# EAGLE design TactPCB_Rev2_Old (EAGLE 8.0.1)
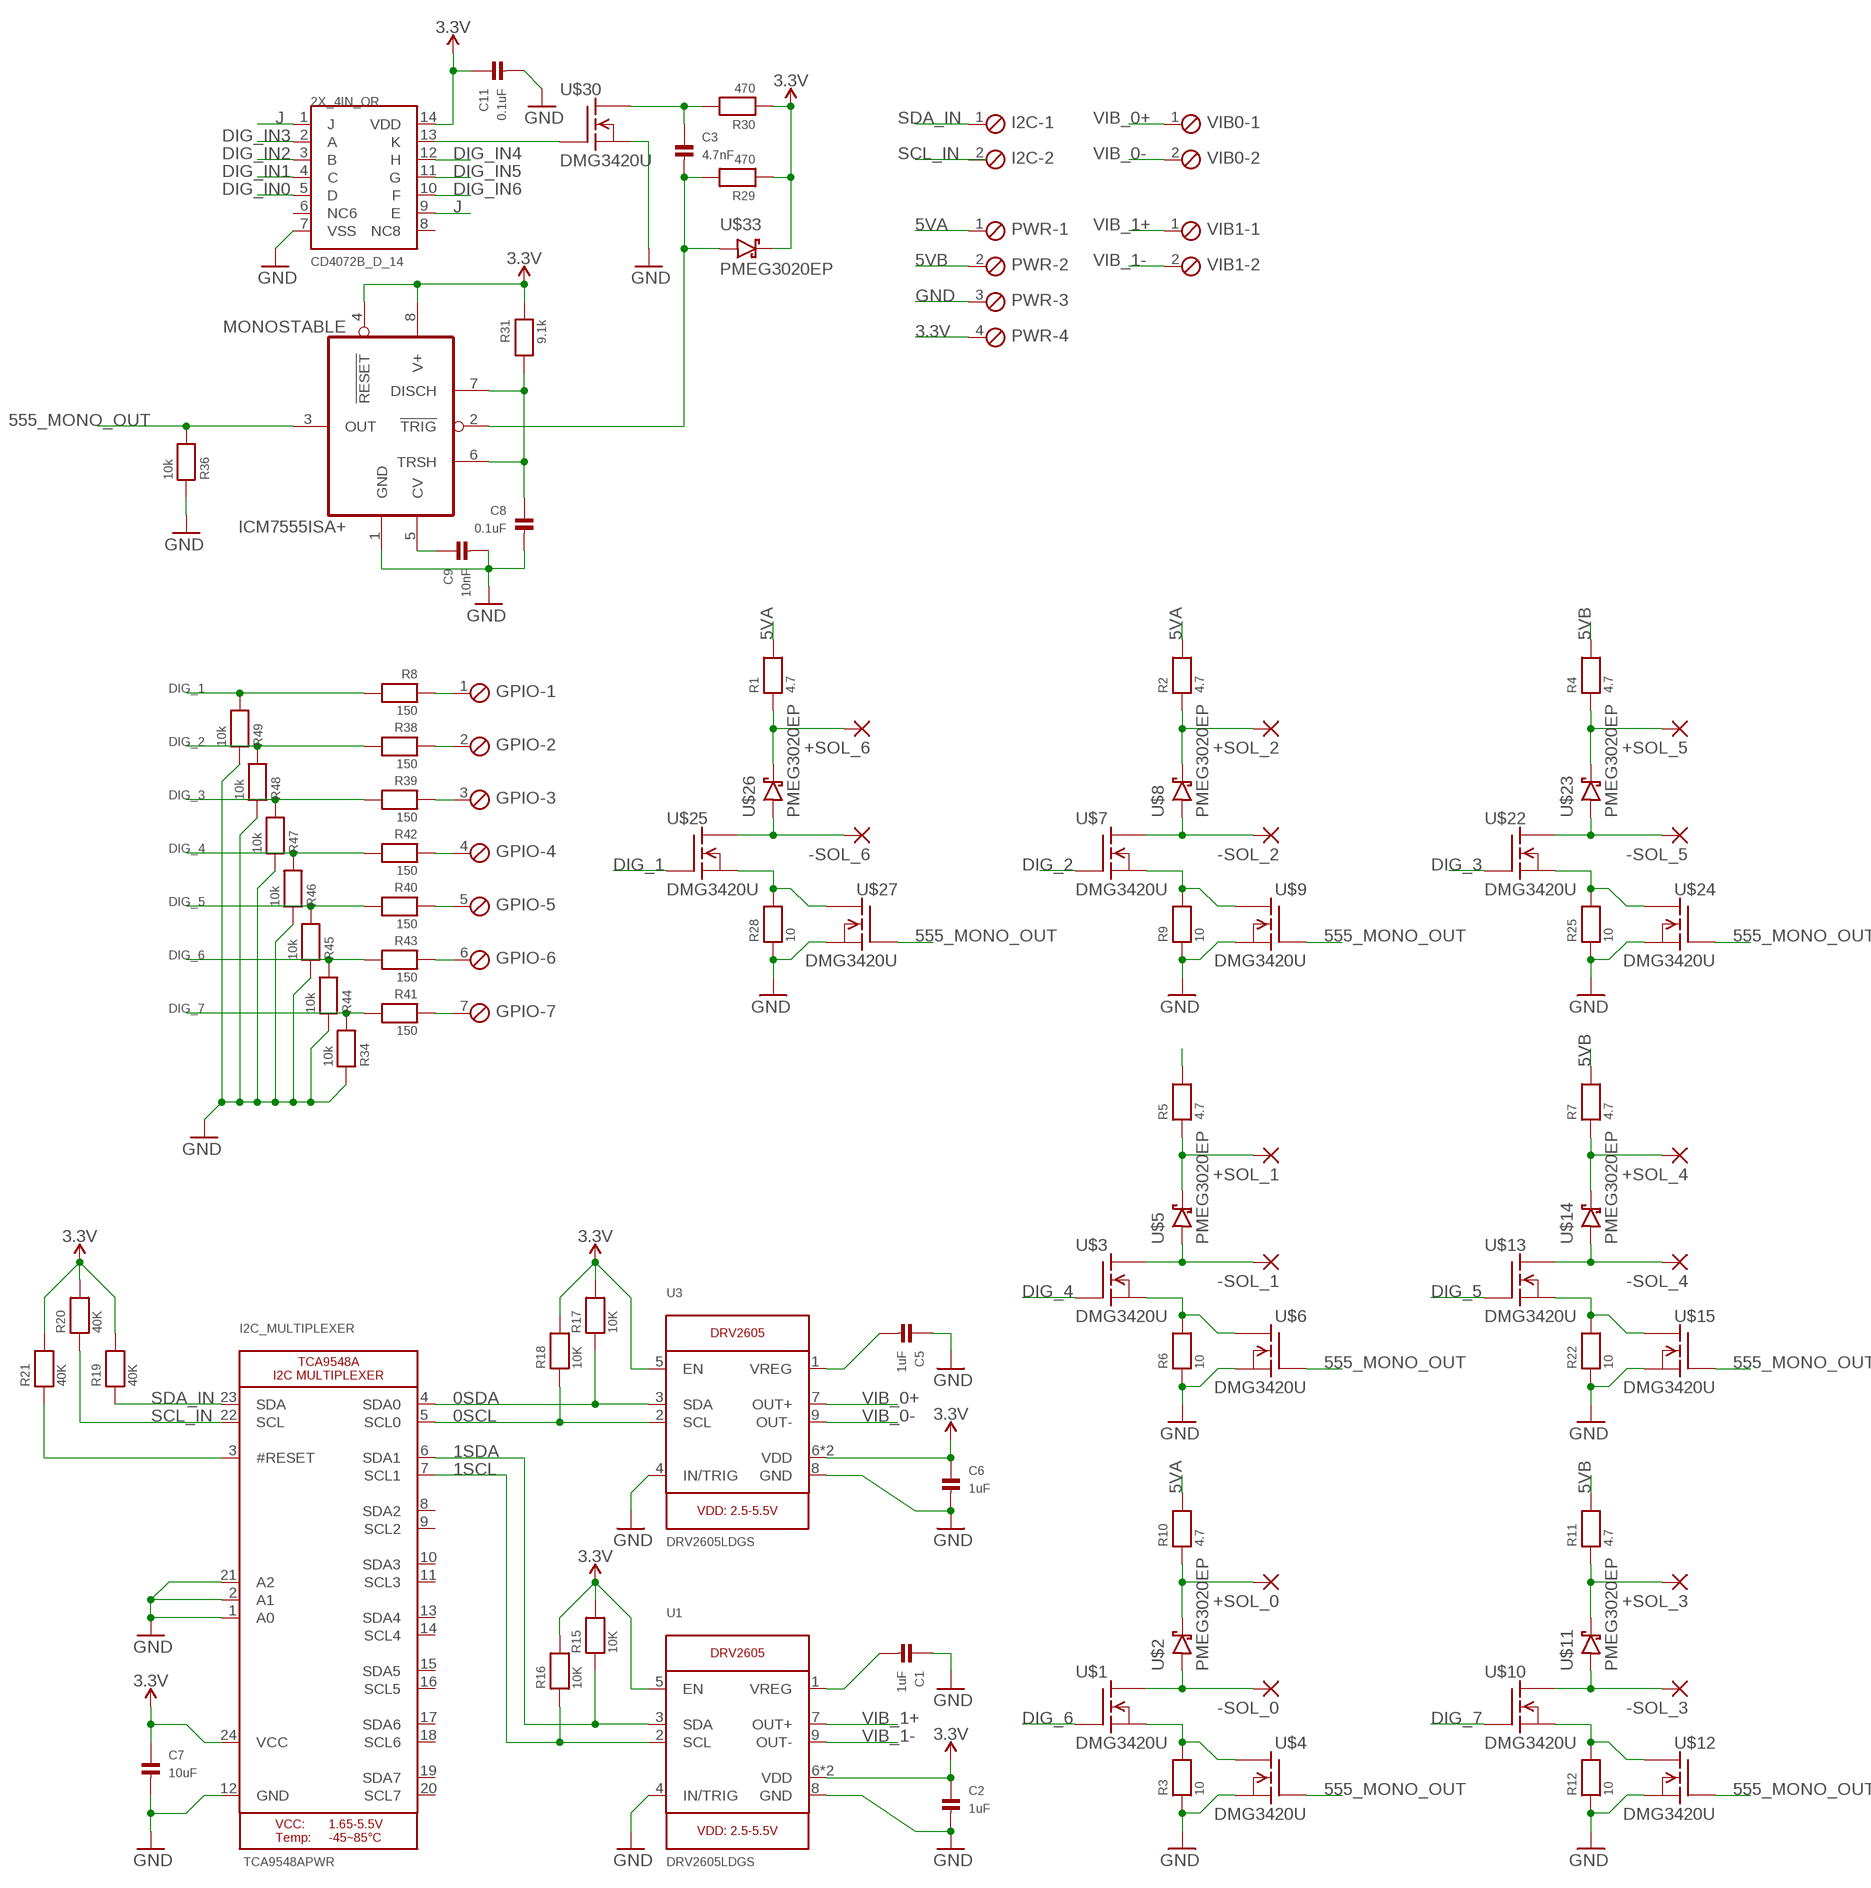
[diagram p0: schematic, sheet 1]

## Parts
2X_4IN_OR  CD4072B_D_14  [SOIC-14]
+SOL_0  2,15/1,0  [2,15/1,0]
+SOL_1  2,15/1,0  [2,15/1,0]
+SOL_2  2,15/1,0  [2,15/1,0]
+SOL_3  2,15/1,0  [2,15/1,0]
+SOL_4  2,15/1,0  [2,15/1,0]
+SOL_5  2,15/1,0  [2,15/1,0]
+SOL_6  2,15/1,0  [2,15/1,0]
-SOL_0  2,15/1,0  [2,15/1,0]
-SOL_1  2,15/1,0  [2,15/1,0]
-SOL_2  2,15/1,0  [2,15/1,0]
-SOL_3  2,15/1,0  [2,15/1,0]
-SOL_4  2,15/1,0  [2,15/1,0]
-SOL_5  2,15/1,0  [2,15/1,0]
-SOL_6  2,15/1,0  [2,15/1,0]
C1  1uF  CAP_CERAMIC0805  [0805]
C2  1uF  CAP_CERAMIC0805  [0805]
C3  4.7nF  CAP_CERAMIC0805  [0805]
C5  1uF  CAP_CERAMIC0805  [0805]
C6  1uF  CAP_CERAMIC0805  [0805]
C7  10uF  CAP_CERAMIC0805  [0805]
C8  0.1uF  CAP_CERAMIC0805  [0805]
C9  10nF  CAP_CERAMIC0805  [0805]
C11  0.1uF  CAP_CERAMIC0805  [0805]
GPIO  MPT7  [7POL254]
I2C  MPT2  [2POL254]
I2C_MULTIPLEXER  TCA9548APWR  TCA9548A  [TSSOP24]
MONOSTABLE  ICM7555ISA+  [SOIC-8]
PWR  MPT4  [4POL254]
R1  4.7  RESISTOR0805  [0805]
R2  4.7  RESISTOR0805  [0805]
R3  10  RESISTOR0805  [0805]
R4  4.7  RESISTOR0805  [0805]
R5  4.7  RESISTOR0805  [0805]
R6  10  RESISTOR0805  [0805]
R7  4.7  RESISTOR0805  [0805]
R8  150  RESISTOR0805  [0805]
R9  10  RESISTOR0805  [0805]
R10  4.7  RESISTOR0805  [0805]
R11  4.7  RESISTOR0805  [0805]
R12  10  RESISTOR0805  [0805]
R15  10K  RESISTOR0805  [0805]
R16  10K  RESISTOR0805  [0805]
R17  10K  RESISTOR0805  [0805]
R18  10K  RESISTOR0805  [0805]
R19  40K  RESISTOR0805  [0805]
R20  40K  RESISTOR0805  [0805]
R21  40K  RESISTOR0805  [0805]
R22  10  RESISTOR0805  [0805]
R25  10  RESISTOR0805  [0805]
R28  10  RESISTOR0805  [0805]
R29  470  RESISTOR0805  [0805]
R30  470  RESISTOR0805  [0805]
R31  9.1k  RESISTOR0805  [0805]
R34  10k  RESISTOR0805  [0805]
R36  10k  RESISTOR0805  [0805]
R38  150  RESISTOR0805  [0805]
R39  150  RESISTOR0805  [0805]
R40  150  RESISTOR0805  [0805]
R41  150  RESISTOR0805  [0805]
R42  150  RESISTOR0805  [0805]
R43  150  RESISTOR0805  [0805]
R44  10k  RESISTOR0805  [0805]
R45  10k  RESISTOR0805  [0805]
R46  10k  RESISTOR0805  [0805]
R47  10k  RESISTOR0805  [0805]
R48  10k  RESISTOR0805  [0805]
R49  10k  RESISTOR0805  [0805]
U1  DRV2605LDGS  DRV2605_SOP  [PSOP10]
U3  DRV2605LDGS  DRV2605_SOP  [PSOP10]
U$1  DMG3420U  [SOT23-3]
U$2  PMEG3020EP  [SOD128]
U$3  DMG3420U  [SOT23-3]
U$4  DMG3420U  [SOT23-3]
U$5  PMEG3020EP  [SOD128]
U$6  DMG3420U  [SOT23-3]
U$7  DMG3420U  [SOT23-3]
U$8  PMEG3020EP  [SOD128]
U$9  DMG3420U  [SOT23-3]
U$10  DMG3420U  [SOT23-3]
U$11  PMEG3020EP  [SOD128]
U$12  DMG3420U  [SOT23-3]
U$13  DMG3420U  [SOT23-3]
U$14  PMEG3020EP  [SOD128]
U$15  DMG3420U  [SOT23-3]
U$22  DMG3420U  [SOT23-3]
U$23  PMEG3020EP  [SOD128]
U$24  DMG3420U  [SOT23-3]
U$25  DMG3420U  [SOT23-3]
U$26  PMEG3020EP  [SOD128]
U$27  DMG3420U  [SOT23-3]
U$30  DMG3420U  [SOT23-3]
U$33  PMEG3020EP  [SOD128]
VIB0  MPT2  [2POL254]
VIB1  MPT2  [2POL254]

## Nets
0SCL: I2C_MULTIPLEXER.5(SCL0) R18.1 U3.2(SCL)
0SDA: I2C_MULTIPLEXER.4(SDA0) R17.1 U3.3(SDA)
1SCL: I2C_MULTIPLEXER.7(SCL1) R16.1 U1.2(SCL)
1SDA: I2C_MULTIPLEXER.6(SDA1) R15.1 U1.3(SDA)
3.3V: 2X_4IN_OR.14(VDD) C2.1 C6.1 C7.1 C11.1 I2C_MULTIPLEXER.24(VCC) MONOSTABLE.4(!RESET) MONOSTABLE.8(V+) PWR.4 R15.2 R16.2 R17.2 R18.2 R19.2 R20.2 R21.2 R29.1 R30.1 R31.1 U1.5(EN) U1.6(VDD) U1.10(VDD) U3.5(EN) U3.6(VDD) U3.10(VDD) U$33.2
5V_PWM: +SOL_0.1(P) +SOL_1.1(P) +SOL_2.1(P) +SOL_3.1(P) +SOL_4.1(P) +SOL_5.1(P) +SOL_6.1(P) R1.1 R2.1 R4.1 R5.1 R7.1 R10.1 R11.1 U$2.2 U$5.2 U$8.2 U$11.2 U$14.2 U$23.2 U$26.2
5VA: PWR.1 R1.2 R2.2 R5.2 R10.2
5VB: PWR.2 R4.2 R7.2 R11.2
555_MONO_OUT: MONOSTABLE.3(OUT) R36.2 U$4.1(G) U$6.1(G) U$9.1(G) U$12.1(G) U$15.1(G) U$24.1(G) U$27.1(G)
DIG_1: R8.2 R49.2 U$25.1(G)
DIG_2: R38.2 R48.2 U$7.1(G)
DIG_3: R39.2 R47.2 U$22.1(G)
DIG_4: R42.2 R46.2 U$3.1(G)
DIG_5: R40.2 R45.2 U$13.1(G)
DIG_6: R43.2 R44.2 U$1.1(G)
DIG_7: R34.2 R41.2 U$10.1(G)
DIG_IN0: 2X_4IN_OR.5(D)
DIG_IN1: 2X_4IN_OR.4(C)
DIG_IN2: 2X_4IN_OR.3(B)
DIG_IN3: 2X_4IN_OR.2(A)
DIG_IN4: 2X_4IN_OR.12(H)
DIG_IN5: 2X_4IN_OR.11(G)
DIG_IN6: 2X_4IN_OR.10(F)
DIG_IN8: GPIO.2 R38.1
DIG_IN9: GPIO.4 R42.1
DIG_IN10: GPIO.6 R43.1
GND: 2X_4IN_OR.7(VSS) C1.1 C2.2 C5.1 C6.2 C7.2 C8.2 C9.2 C11.2 I2C_MULTIPLEXER.1(A0) I2C_MULTIPLEXER.2(A1) I2C_MULTIPLEXER.12(GND) I2C_MULTIPLEXER.21(A2) MONOSTABLE.1(GND) PWR.3 R3.1 R6.1 R9.1 R12.1 R22.1 R25.1 R28.1 R34.1 R36.1 R44.1 R45.1 R46.1 R47.1 R48.1 R49.1 U1.4(IN/TRIG) U1.8(GND) U3.4(IN/TRIG) U3.8(GND) U$4.3(S) U$6.3(S) U$9.3(S) U$12.3(S) U$15.3(S) U$24.3(S) U$27.3(S) U$30.3(S)
J: 2X_4IN_OR.1(J) 2X_4IN_OR.9(E)
N$1: R3.2 U$1.3(S) U$4.2(D)
N$3: -SOL_0.1(P) U$1.2(D) U$2.1
N$5: -SOL_1.1(P) U$3.2(D) U$5.1
N$6: R6.2 U$3.3(S) U$6.2(D)
N$8: -SOL_2.1(P) U$7.2(D) U$8.1
N$9: R9.2 U$7.3(S) U$9.2(D)
N$11: -SOL_3.1(P) U$10.2(D) U$11.1
N$12: R12.2 U$10.3(S) U$12.2(D)
N$14: -SOL_4.1(P) U$13.2(D) U$14.1
N$15: C1.2 U1.1(VREG)
N$16: C5.2 U3.1(VREG)
N$17: C3.1 R30.2 U$30.2(D)
N$18: C3.2 MONOSTABLE.2(!TRIG) R29.2 U$33.1
N$23: R22.2 U$13.3(S) U$15.2(D)
N$25: -SOL_5.1(P) U$22.2(D) U$23.1
N$26: R25.2 U$22.3(S) U$24.2(D)
N$28: -SOL_6.1(P) U$25.2(D) U$26.1
N$29: R28.2 U$25.3(S) U$27.2(D)
N$32: C9.1 MONOSTABLE.5(CV)
N$33: C8.1 MONOSTABLE.6(TRSH) MONOSTABLE.7(DISCH) R31.2
N$34: 2X_4IN_OR.13(K) U$30.1(G)
N$41: GPIO.1 R8.1
N$46: GPIO.7 R41.1
N$47: GPIO.3 R39.1
N$48: GPIO.5 R40.1
RESET: I2C_MULTIPLEXER.3(#RESET) R21.1
SCL_IN: I2C.2 I2C_MULTIPLEXER.22(SCL) R20.1
SDA_IN: I2C.1 I2C_MULTIPLEXER.23(SDA) R19.1
VIB_0+: U3.7(OUT+) VIB0.1
VIB_0-: U3.9(OUT-) VIB0.2
VIB_1+: U1.7(OUT+) VIB1.1
VIB_1-: U1.9(OUT-) VIB1.2
Unconnected: 2X_4IN_OR.6(NC6) 2X_4IN_OR.8(NC8) I2C_MULTIPLEXER.8(SDA2) I2C_MULTIPLEXER.9(SCL2) I2C_MULTIPLEXER.10(SDA3) I2C_MULTIPLEXER.11(SCL3) I2C_MULTIPLEXER.13(SDA4) I2C_MULTIPLEXER.14(SCL4) I2C_MULTIPLEXER.15(SDA5) I2C_MULTIPLEXER.16(SCL5) I2C_MULTIPLEXER.17(SDA6) I2C_MULTIPLEXER.18(SCL6) I2C_MULTIPLEXER.19(SDA7) I2C_MULTIPLEXER.20(SCL7)

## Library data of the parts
2X_4IN_OR = SD2017_StephenMiles:CD4072B_D_14
+SOL_0 +SOL_1-+SOL_6 -SOL_0 -SOL_1--SOL_6 = wirepad:2,15/1,0: THROUGH-HOLE PAD
C1-C3 C5-C9 C11 = microbuilder:CAP_CERAMIC: Ceramic Capacitors
GPIO = con-phoenix-254:MPT7: PHOENIX CONNECTOR; OC_FARNELL: unknown; OC_NEWARK: unknown
I2C VIB0 VIB1 = con-phoenix-254:MPT2: PHOENIX CONNECTOR; OC_FARNELL: unknown; OC_NEWARK: unknown
I2C_MULTIPLEXER = TactilePCB:TCA9548A: TCA9548A I2C Multiplexer
MONOSTABLE = SD2017_StephenMiles:ICM7555ISA+
PWR = con-phoenix-254:MPT4: PHOENIX CONNECTOR; OC_FARNELL: unknown; OC_NEWARK: unknown
R1-R12 R15-R22 R25 R28-R31 R34 R36 R38-R49 = microbuilder:RESISTOR: Resistors
U1 U3 = TactilePCB:DRV2605: DRV2605 - Haptic Driver for ERM/LRA Motors
U$1 U$3 U$4 U$6 U$7 U$9 U$10 U$12 U$13 U$15 U$22 U$24 U$25 U$27 U$30 = SD2017_StephenMiles:DMG3420U: N-Channel MosFET 20Vds, 1Vgs(th), 5.47A Id
U$2 U$5 U$8 U$11 U$14 U$23 U$26 U$33 = SD2017_StephenMiles:PMEG3020EP: Schottky Diode

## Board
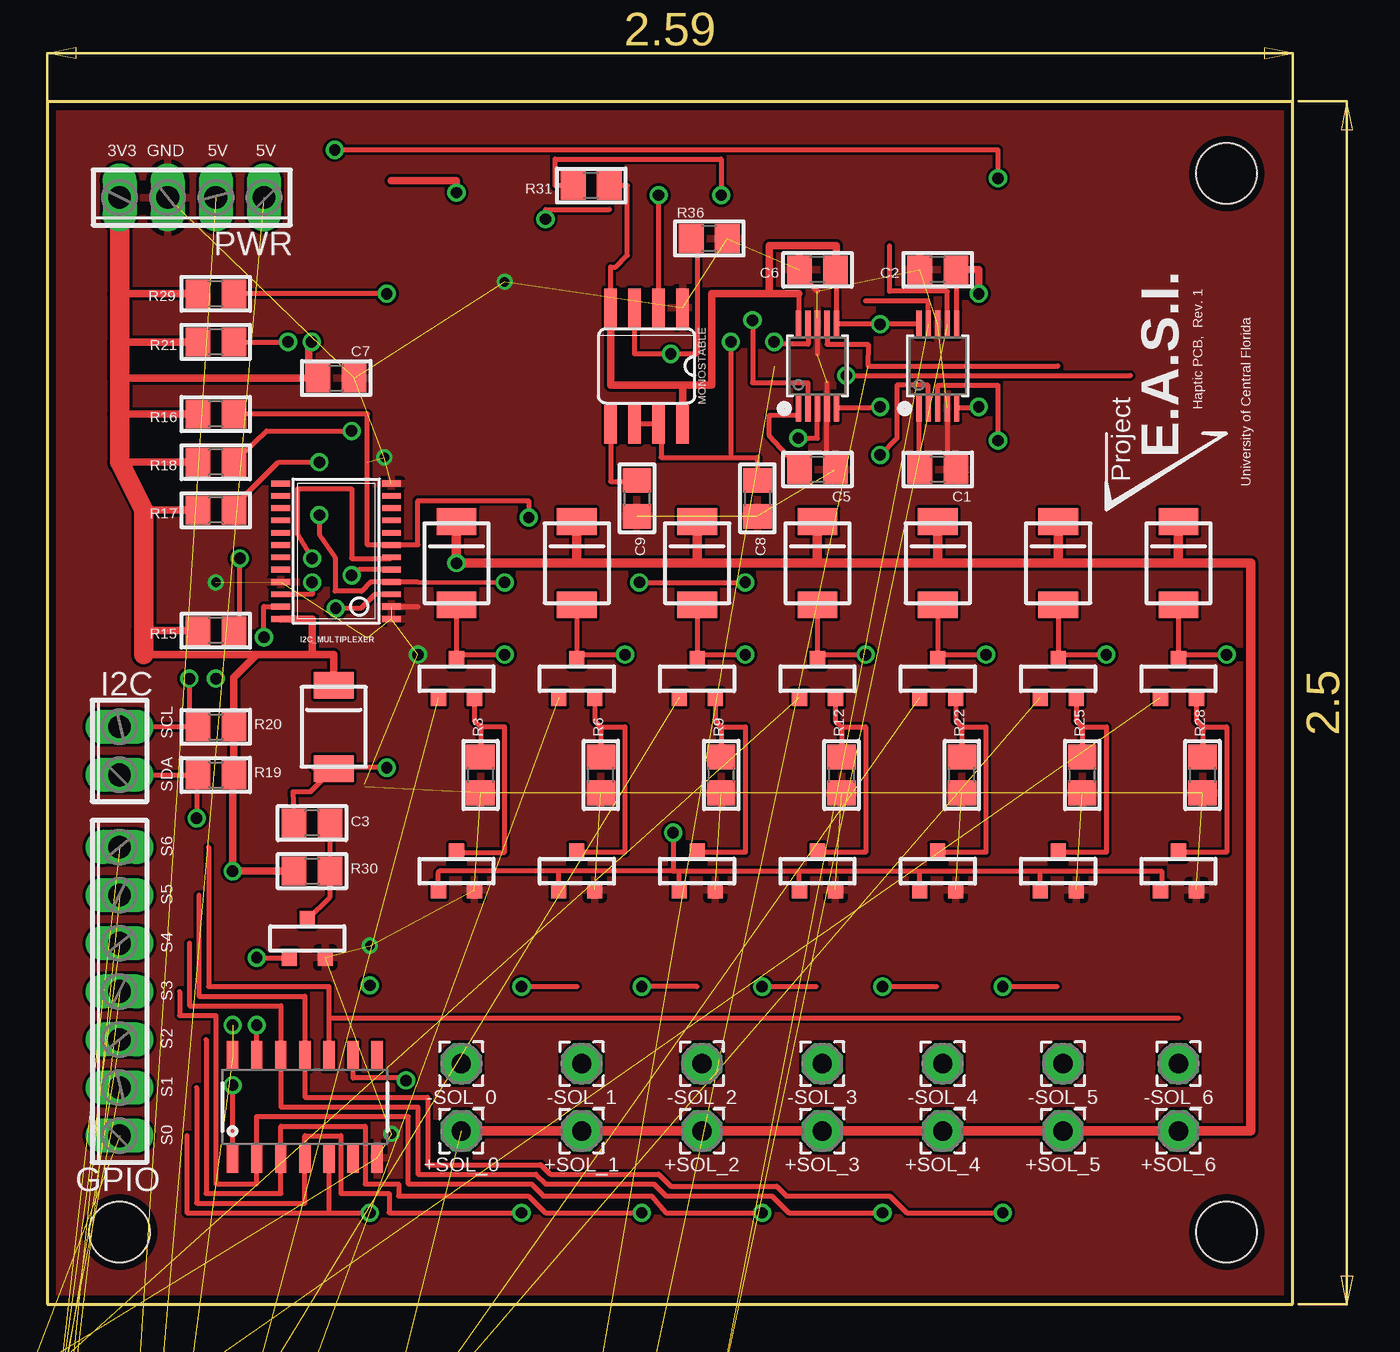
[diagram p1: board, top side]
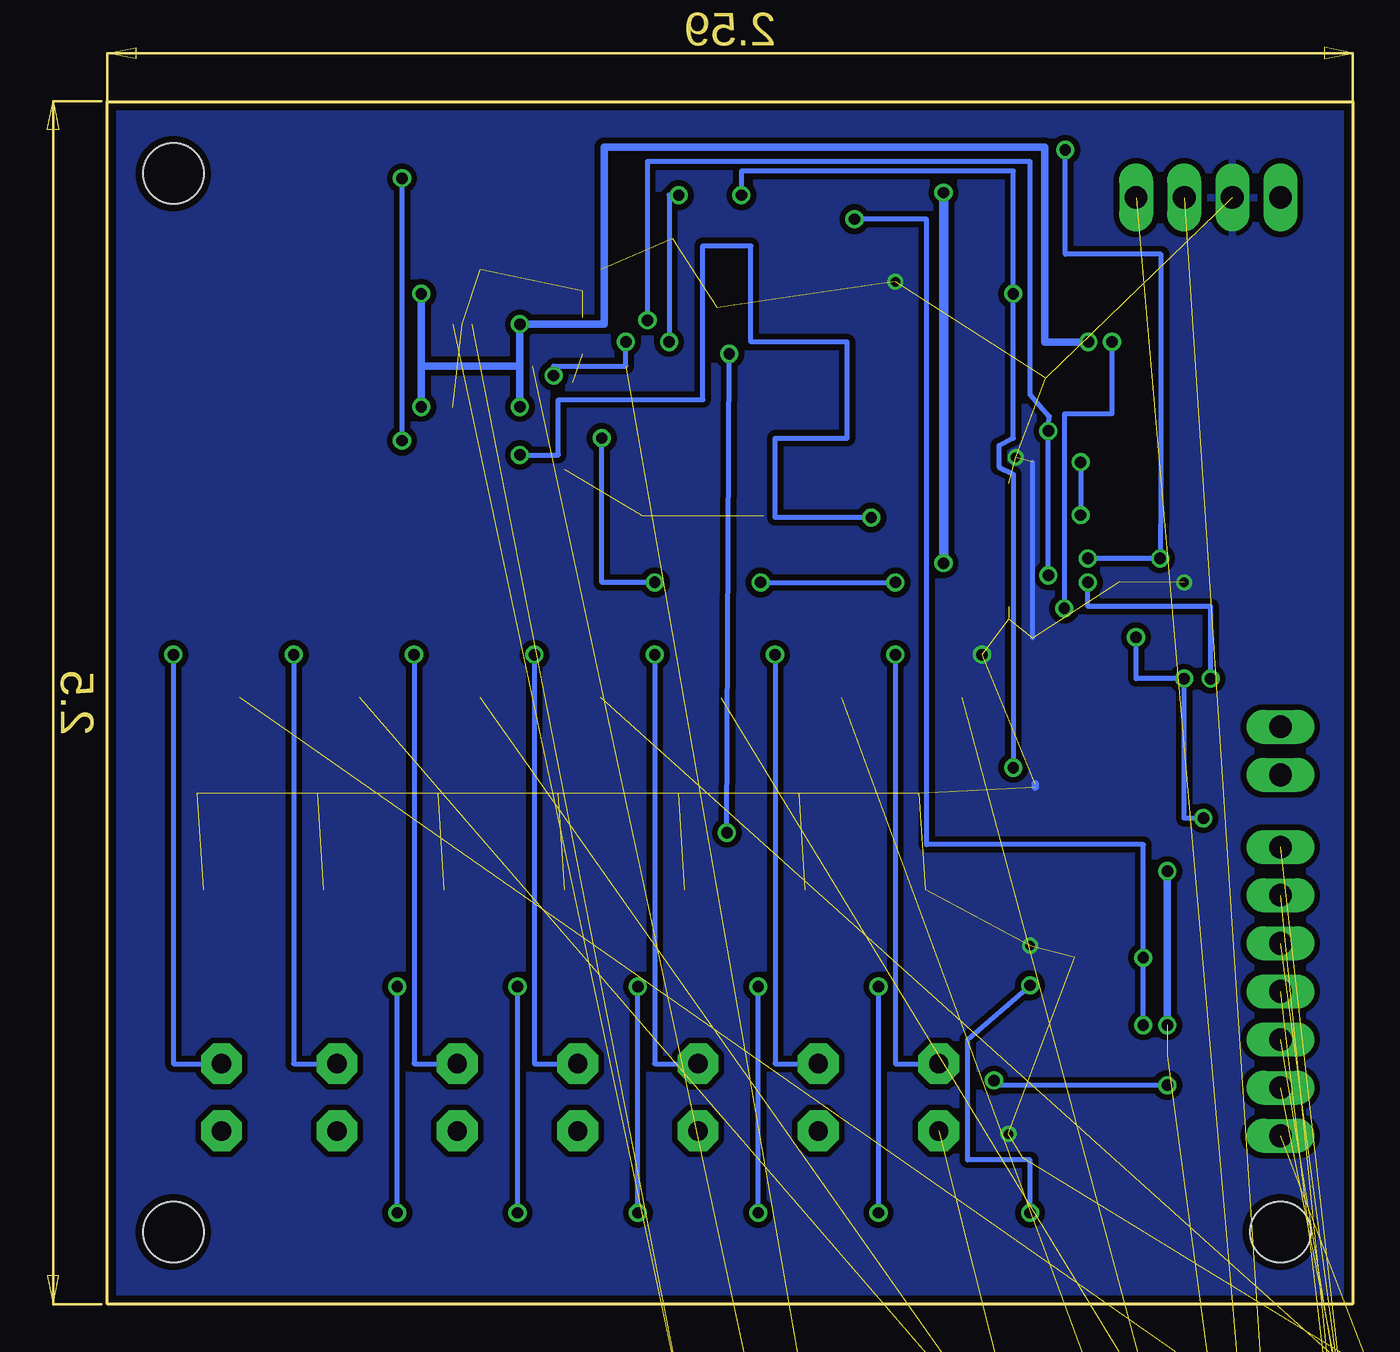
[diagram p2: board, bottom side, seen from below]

Size 68.88 x 66.35 mm. Coordinates in mm from the lower left corner, seen from the top.
Outline: 0,0 65.71,0 65.71,63.49 0,63.49 0,0
Copper layers (1*16): Top 0.0356mm / dielectric 1.5011mm / Bottom 0.0356mm
Design rules "oshpark-2layer": minimum track width 6mil, minimum drill 13mil, track to track 6mil, track to pad 6mil, pad to pad 6mil, via to via 6mil, smd to smd 6mil, copper to edge 15mil, drill to drill 6mil, minimum pad ring 7mil, minimum via ring 7mil, stop-mask expansion 2.5mil, vias tented up to drill 0mil, thermal gap 10mil
Holes 3.2 mm at 62.23,59.69 62.23,3.81 3.81,3.81

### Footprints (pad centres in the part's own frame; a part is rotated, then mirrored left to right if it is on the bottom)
SOIC-14 = smd 0.6 x 1.55: 1 -3.81,-2.7; 2 -2.54,-2.7; 3 -1.27,-2.7; 4 0,-2.7; 5 1.27,-2.7; 6 2.54,-2.7; 7 3.81,-2.7; 8 3.81,2.7; 9 2.54,2.7; 10 1.27,2.7; 11 0,2.7; 12 -1.27,2.7; 13 -2.54,2.7; 14 -3.81,2.7
2,15/1,0 = drill 1.016 pad 2.159 octagon: 1 0,0
0805 = smd 1.3 x 1.5: 1 -0.95,0; 2 0.95,0
7POL254 = drill 1.2 long: 1 -7.62,0; 2 -5.08,0; 3 -2.54,0; 4 0,0; 5 2.54,0; 6 5.08,0; 7 7.62,0
2POL254 = drill 1.2 long: 1 -1.27,0; 2 1.27,0
TSSOP24 = smd 0.305 x 0.991: 1 -3.575,-2.918; 2 -2.925,-2.918; 3 -2.275,-2.918; 4 -1.625,-2.918; 5 -0.975,-2.918; 6 -0.325,-2.918; 7 0.325,-2.918; 8 0.975,-2.918; 9 1.625,-2.918; 10 2.275,-2.918; 11 2.925,-2.918; 12 3.575,-2.918; 13 3.575,2.918; 14 2.925,2.918; 15 2.275,2.918; 16 1.625,2.918; 17 0.975,2.918; 18 0.325,2.918; 19 -0.325,2.918; 20 -0.975,2.918; 21 -1.625,2.918; 22 -2.275,2.918; 23 -2.925,2.918; 24 -3.575,2.918
SOIC-8 = smd 0.66 x 2.032: 1 -1.905,-3.073; 2 -0.635,-3.073; 3 0.635,-3.073; 4 1.905,-3.073; 5 1.905,3.073; 6 0.635,3.073; 7 -0.635,3.073; 8 -1.905,3.073
4POL254 = drill 1.2 long: 1 -3.81,0; 2 -1.27,0; 3 1.27,0; 4 3.81,0
PSOP10 = smd 0.28 x 1.45: 1 -1,-2.2; 2 -0.5,-2.2; 3 0,-2.2; 4 0.5,-2.2; 5 1,-2.2; 6 1,2.2; 7 0.5,2.2; 8 0,2.2; 9 -0.5,2.2; 10 -1,2.2
SOT23-3 = smd 0.8 x 0.9: 1 -0.95,-1; 2 0,1; 3 0.95,-1
SOD128 = smd 1.4 x 2.1: 1 -2.2,0; 2 2.2,0

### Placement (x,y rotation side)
2X_4IN_OR  13.59,10.41 0 top
+SOL_0  21.84,9.14 180 top
+SOL_1  28.19,9.14 180 top
+SOL_2  34.54,9.14 180 top
+SOL_3  40.89,9.14 180 top
+SOL_4  47.24,9.14 180 top
+SOL_5  53.59,9.14 180 top
+SOL_6  59.69,9.14 180 top
-SOL_0  21.84,12.7 180 top
-SOL_1  28.19,12.7 180 top
-SOL_2  34.54,12.7 180 top
-SOL_3  40.89,12.7 180 top
-SOL_4  47.24,12.7 180 top
-SOL_5  53.59,12.7 180 top
-SOL_6  59.69,12.7 180 top
C1  46.99,44.07 180 top
C2  46.99,54.61 180 top
C3  13.97,25.4 180 top
C5  40.64,44.07 180 top
C6  40.64,54.61 180 top
C7  15.24,48.9 0 top
C8  37.47,42.55 270 top
C9  31.11,42.55 270 top
C11  not placed on the board
GPIO  3.81,16.51 90 top
I2C  3.81,29.21 90 top
I2C_MULTIPLEXER  15.24,39.75 90 top
MONOSTABLE  31.62,49.53 180 top
PWR  7.62,58.42 180 top
R1  not placed on the board
R2  not placed on the board
R3  22.86,27.94 90 top
R4  not placed on the board
R5  not placed on the board
R6  29.21,27.94 90 top
R7  not placed on the board
R8  not placed on the board
R9  35.56,27.94 90 top
R10  not placed on the board
R11  not placed on the board
R12  41.91,27.94 90 top
R15  8.89,35.56 180 top
R16  8.89,46.99 180 top
R17  8.89,41.91 180 top
R18  8.89,44.45 180 top
R19  8.89,27.94 0 top
R20  8.89,30.48 0 top
R21  8.89,50.8 180 top
R22  48.26,27.94 90 top
R25  54.61,27.94 90 top
R28  60.96,27.94 90 top
R29  8.89,53.34 0 top
R30  13.97,22.86 0 top
R31  28.7,59.05 180 top
R34  not placed on the board
R36  34.92,56.26 180 top
R38  not placed on the board
R39  not placed on the board
R40  not placed on the board
R41  not placed on the board
R42  not placed on the board
R43  not placed on the board
R44  not placed on the board
R45  not placed on the board
R46  not placed on the board
R47  not placed on the board
R48  not placed on the board
R49  not placed on the board
U1  46.99,49.53 0 top
U3  40.64,49.53 0 top
U$1  21.59,33.02 0 top
U$2  21.59,39.12 90 top
U$3  27.94,33.02 0 top
U$4  21.59,22.86 0 top
U$5  27.94,39.12 90 top
U$6  27.94,22.86 0 top
U$7  34.29,33.02 0 top
U$8  34.29,39.12 90 top
U$9  34.29,22.86 0 top
U$10  40.64,33.02 0 top
U$11  40.64,39.12 90 top
U$12  40.64,22.86 0 top
U$13  46.99,33.02 0 top
U$14  46.99,39.12 90 top
U$15  46.99,22.86 0 top
U$22  53.34,33.02 0 top
U$23  53.34,39.12 90 top
U$24  53.34,22.86 0 top
U$25  59.69,33.02 0 top
U$26  59.69,39.12 90 top
U$27  59.69,22.86 0 top
U$30  13.72,19.3 0 top
U$33  15.11,30.48 90 top
VIB0  not placed on the board
VIB1  not placed on the board

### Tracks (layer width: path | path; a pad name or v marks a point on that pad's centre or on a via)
0SCL  (via drill 0.6)
  Top 0.254: 9.84,44.89 R18.1 11.56,46.1 v16.05,46.1 | I2C_MULTIPLEXER.5 16.42,38.78 v16.05,38.48 | 40.13,47.47 U3.2 40.13,48.64 37.21,48.64 v37.21,51.94
  Bottom 0.254: v16.05,38.48 v16.05,46.1 16,46.86 17.02,48.01 17.02,60.33 37.21,60.33 v37.21,51.94
0SDA  (via drill 0.6)
  Top 0.254: v24.13,38.1 19.53,38.13 I2C_MULTIPLEXER.4 17.04,38.13 16.59,37.64 15.19,37.64 15.19,39.42 14.35,40.64 v14.35,41.66 | v39.62,45.72 40.64,45.72 U3.3 | R17.1 9.84,42.1 12.19,44.45 v14.35,44.45 | v31.24,38.1 v36.83,38.1
  Bottom 0.254: v31.24,38.1 v24.13,38.1 | v36.83,38.1 39.62,38.1 v39.62,45.72 | v14.35,44.45 v14.35,41.66
1SCL  (via drill 0.6)
  Top 0.254: R16.1 16.89,46.99 16.89,40.08 I2C_MULTIPLEXER.7 19.56,40.08 19.56,42.42 25.4,42.42 v25.4,41.53 | U1.2 46.48,48.51 44.83,48.51 44.83,45.72 v43.94,44.83
  Bottom 0.254: v25.4,41.53 30.48,41.53 30.48,45.72 26.67,45.72 26.67,50.8 31.75,50.8 31.75,55.88 34.29,55.88 34.29,47.75 41.91,47.75 41.91,44.83 v43.94,44.83
1SDA  (via drill 0.6)
  Top 0.254: R15.1 10.16,35.56 v10.16,39.37 | I2C_MULTIPLEXER.6 18.1,39.37 16.05,39.37 16.05,43.05 13.21,43.05 13.21,40.64 v13.97,39.37 | U1.3 46.99,48.51 50.16,48.51 v50.16,45.59 | v15.16,60.94 50.16,60.94 v50.16,59.44
  Bottom 0.254: v13.97,39.37 v10.16,39.37 10.13,39.37 10.13,40.16 10.11,42.22 10.11,55.42 15.16,55.42 v15.16,60.94 | v50.16,45.59 v50.16,59.44
3.3V  (via drill 0.6)  (2 unrouted)
  Top 0.254: 39.64,53.34 U3.10 | U1.6 47.99,54.61 | U3.5 43.94,47.33 | U1.5 49.15,47.33 | 41.64,54.61 U3.6 v43.94,51.73 U1.10 | R31.1 30.61,59.05 30.61,55.37 29.99,54.75 29.72,54.75 MONOSTABLE.4
  Top 0.406: 5.08,35.56 R15.2 | 5.08,41.91 R17.2 | 3.81,44.45 R18.2 | 3.81,46.99 R16.2 | R21.2 3.81,50.8 | R29.1 3.81,53.34 | 33.53,48.51 35.05,48.51 35.05,53.34 38.1,53.34 | 33.53,48.51 29.72,48.51 MONOSTABLE.4 | 47.99,54.61 C2.1 49.15,54.61 v49.15,53.34 | 38.1,53.34 39.64,53.34 | 5.08,34.29 11.05,34.29 | 11.05,34.29 9.84,33.08 R20.2 R19.2 9.78,27.88 v9.78,22.86 R30.1 | 43.94,47.33 v43.94,47.37 | 49.15,47.33 v49.15,47.37 | 38.1,53.34 38.1,55.88 41.64,55.88 41.64,54.61 C6.1 | 13.97,34.29 13.97,36.18 I2C_MULTIPLEXER.24 | 13.97,34.29 15.11,34.29 U$33.2 | 11.05,34.29 13.97,34.29 | 13.79,48.9 C7.1 | 13.79,48.9 3.81,48.9 | v13.95,50.8 13.79,50.8 13.79,48.9 | 33.53,48.51 MONOSTABLE.8
  Top 1.016: 5.08,34.29 5.08,35.56 5.08,41.91 3.81,44.45 3.81,46.99 3.81,48.9 3.81,50.8 3.81,53.34 PWR.4
  Bottom 0.406: v9.78,14.73 v9.78,22.86 | v43.94,47.37 43.94,49.53 | 43.94,49.53 v43.94,51.73 39.5,51.73 39.5,61.09 16.26,61.09 16.26,50.8 v13.95,50.8 | 49.15,49.53 v49.15,47.37 | 49.15,49.53 v49.15,53.34 | 43.94,49.53 49.15,49.53
5V_PWM  (via drill 0.6)  (7 unrouted)
  Top 0.406: v21.59,58.67 21.59,59.31 18.14,59.31
  Top 0.508: U$2.2 v21.59,39.12 27.94,39.12 | 27.94,39.12 U$5.2 | 27.94,39.12 34.29,39.12 | 34.29,39.12 U$8.2 | 34.29,39.12 40.64,39.12 | 40.64,39.12 U$11.2 | 40.64,39.12 46.99,39.12 | 46.99,39.12 U$14.2 | 46.99,39.12 53.34,39.12 | 53.34,39.12 U$23.2 | 53.34,39.12 59.69,39.12 | 59.69,39.12 U$26.2 | 59.69,39.12 63.5,39.12 63.5,9.14 +SOL_6.1 +SOL_5.1 +SOL_4.1 +SOL_3.1 +SOL_2.1 +SOL_1.1 +SOL_0.1
  Bottom 0.508: v21.59,58.67 v21.59,39.12
5VA  (4 unrouted)
5VB  (3 unrouted)
555_MONO_OUT  (via drill 0.6)
  Top 0.254: U$4.1 20.64,22.8 20.7,22.86 26.99,22.86 | 46.04,22.86 52.39,22.86 | 39.69,22.86 46.04,22.86 | 33.34,22.86 39.69,22.86 | 33.02,22.86 33.34,22.86 | 33.02,22.86 26.99,22.86 | 52.39,22.86 58.8,22.86 58.8,21.92 U$27.1 | U$24.1 52.39,22.86 | U$15.1 46.04,22.86 | U$12.1 39.69,22.86 | U$9.1 33.34,22.86 | U$6.1 26.99,22.86 | v33.02,24.89 33.02,22.86 | MONOSTABLE.3 30.99,50.16 v32.89,50.16 34.29,50.16 34.29,55.56 R36.2
  Bottom 0.254: v33.02,24.89 v32.89,50.16
DIG_1  (2 unrouted)
DIG_2  (2 unrouted)
DIG_3  (2 unrouted)
DIG_4  (2 unrouted)
DIG_5  (2 unrouted)
DIG_6  (2 unrouted)
DIG_7  (2 unrouted)
DIG_IN0  (via drill 0.6)
  Top 0.254: 7.37,8.89 7.37,4.83 14.86,4.83 | 2X_4IN_OR.5 14.86,4.83 | 14.86,4.83 v17.02,4.83
  Bottom 0.254: v17.02,4.83 17.02,7.62 20.32,7.62 20.32,13.97 v17.02,16.83
DIG_IN1  (via drill 0.6)
  Top 0.254: 7.87,11.43 7.87,5.33 13.59,5.33 2X_4IN_OR.4 13.59,8.89 15.49,8.89 15.49,5.84 18.03,5.84 18.03,4.83 v25.02,4.83 | v25.02,16.76 27.94,16.76
  Bottom 0.254: v25.02,4.83 v25.02,16.76
DIG_IN2  (via drill 0.6)
  Top 0.254: 8.38,13.97 8.38,5.84 12.32,5.84 2X_4IN_OR.3 12.32,9.4 16.76,9.4 16.76,6.35 18.54,6.35 18.54,5.71 25.38,5.71 26.26,4.83 v31.37,4.83 | 34.29,16.76 v31.37,16.76
  Bottom 0.254: v31.37,4.83 v31.37,16.76
DIG_IN3  (via drill 0.6)
  Top 0.254: 6.99,16.51 6.99,15.24 8.89,15.24 8.89,6.35 11.05,6.35 2X_4IN_OR.2 11.05,9.91 19.05,9.91 19.05,6.35 25.53,6.35 26.16,5.71 31.88,5.71 32.64,4.83 v37.72,4.83 | v37.72,16.76 40.57,16.76
  Bottom 0.254: v37.72,4.83 v37.72,16.76
DIG_IN4  (via drill 0.6)
  Top 0.254: 7.49,19.05 7.49,15.75 12.32,15.75 2X_4IN_OR.12 12.32,10.41 19.56,10.41 19.56,6.86 25.78,6.86 26.29,6.35 32,6.35 32.64,5.71 38.23,5.71 39.12,4.83 v44.07,4.83 | v44.07,16.76 46.92,16.76
  Bottom 0.254: v44.07,4.83 v44.07,16.76
DIG_IN5  (via drill 0.6)
  Top 0.254: 8,21.59 8,16.26 13.59,16.26 2X_4IN_OR.11 13.59,10.92 20.07,10.92 20.07,7.37 26.04,7.37 26.54,6.86 32.26,6.86 32.89,6.22 38.48,6.22 38.99,5.71 44.45,5.71 45.34,4.83 v50.42,4.83 | v50.42,16.76 53.27,16.76
  Bottom 0.254: v50.42,4.83 v50.42,16.76
DIG_IN6
  Top 0.254: 8.51,24.13 8.51,16.76 14.86,16.76 14.86,15.11 | 14.86,15.11 2X_4IN_OR.10 | 14.86,15.11 59.69,15.11
DIG_IN8  (1 unrouted)
DIG_IN9  (1 unrouted)
DIG_IN10  (1 unrouted)
GND  (via drill 0.5, 0.6)  (47 unrouted)
  Top 0.254: U1.4 47.49,44.45 C1.1 | C6.2 39.69,54.42 40.64,53.47 | C5.1 41.14,44.9 U3.4 41.15,48.64 | I2C_MULTIPLEXER.2 19.56,36.83 | 18.16,43.31 I2C_MULTIPLEXER.12 | 40.64,52.07 U3.8 40.64,50.16
  Bottom 0.254: 16.89,35.18 16.89,44.45
  Bottom 0.406: 16.74,27.3 16.74,27.46
  other vias: 8.89,38.1 18.16,8.99 17.02,18.92 19.56,34.29 17.78,44.7 24.13,53.98
  pour Top: 0,63.5 0,0 66.04,0 66.04,63.5
  pour Bottom (isolate 0.305): 0,63.5 0,0 66.04,0 66.04,63.5
J  (via drill 0.6)
  Top 0.254: 2X_4IN_OR.1 v9.78,11.56 | v18.92,11.81 18.92,11.94 16.13,11.94 2X_4IN_OR.9
  Bottom 0.254: v9.78,11.56 18.92,11.56 v18.92,11.81
N$1
  Top 0.254: U$1.3 22.54,30.8 22.86,30.48 | 22.86,30.48 R3.2 | U$4.2 24.13,23.86 24.13,30.48 22.86,30.48
N$3  (via drill 0.6)
  Top 0.254: U$2.1 21.59,34.29 | U$1.2 21.59,34.29 | 21.59,34.29 v24.13,34.29
  Bottom 0.254: v24.13,34.29 24.13,12.7 -SOL_0.1
N$5  (via drill 0.6)
  Top 0.254: U$5.1 U$3.2 27.94,34.29 v30.48,34.29
  Bottom 0.254: v30.48,34.29 30.48,12.7 -SOL_1.1
N$6
  Top 0.254: U$3.3 28.89,30.8 29.21,30.48 | 29.21,30.48 R6.2 | 29.21,30.48 30.48,30.48 30.48,23.86 U$6.2
N$8  (via drill 0.6)
  Top 0.254: U$8.1 U$7.2 34.29,34.29 v36.83,34.29
  Bottom 0.254: v36.83,34.29 36.83,12.7 -SOL_2.1
N$9
  Top 0.254: U$7.3 35.24,30.8 35.56,30.48 | 35.56,30.48 R9.2 | 35.56,30.48 36.83,30.48 36.83,23.86 U$9.2
N$11  (via drill 0.6)
  Top 0.254: U$11.1 U$10.2 40.64,34.29 v43.18,34.29
  Bottom 0.254: v43.18,34.29 43.18,12.7 -SOL_3.1
N$12
  Top 0.254: U$10.3 41.59,30.8 41.91,30.48 | 41.91,30.48 R12.2 | 41.91,30.48 43.18,30.48 43.18,23.86 U$12.2
N$14  (via drill 0.6)
  Top 0.254: U$14.1 U$13.2 46.99,34.29 v49.53,34.29
  Bottom 0.254: v49.53,34.29 49.53,12.7 -SOL_4.1
N$15
  Top 0.254: U1.1 45.99,44.5 C1.2
N$16
  Top 0.254: C5.2 39.69,44.13 38.1,45.85 38.1,46.93 39.64,46.93 U3.1
N$17
  Top 0.254: C3.1 R30.2 14.92,21.51 U$30.2
N$18  (via drill 0.6)
  Top 0.254: v17.91,53.34 R29.2 | v17.91,28.32 14.01,28.32 U$33.1 13.88,27.05 12.95,27.05 C3.2 | MONOSTABLE.2 v32.26,58.55
  Bottom 0.254: v17.91,28.32 17.91,43.81 18.67,44.2 18.67,45.34 17.91,45.72 v17.91,53.34 17.91,59.82 32.26,59.82 v32.26,58.55
N$23
  Top 0.254: U$13.3 47.94,30.8 48.26,30.48 | 48.26,30.48 R22.2 | 48.26,30.48 49.53,30.48 49.53,23.86 U$15.2
N$25  (via drill 0.6)
  Top 0.254: U$23.1 U$22.2 arc-90 53.61,34.29 v55.88,34.29
  Bottom 0.254: v55.88,34.29 55.88,12.7 -SOL_5.1
N$26
  Top 0.254: U$22.3 54.29,30.8 54.61,30.48 | 54.61,30.48 R25.2 | 54.61,30.48 55.88,30.48 55.88,23.86 U$24.2
N$28  (via drill 0.6)
  Top 0.254: U$26.1 U$25.2 59.69,34.29 v62.23,34.29
  Bottom 0.254: v62.23,34.29 62.23,12.7 -SOL_6.1
N$29
  Top 0.254: U$25.3 60.64,30.8 60.96,30.48 | 60.96,30.48 R28.2 | 60.96,30.48 62.23,30.48 62.23,23.86 U$27.2
N$32
  Top 0.254: MONOSTABLE.5 29.72,43.43 31.05,43.43 C9.1
N$33  (via drill 0.6)
  Top 0.254: 36.07,44.7 32.38,44.7 32.38,46.46 MONOSTABLE.7 MONOSTABLE.6 | 36.07,44.7 37.47,44.7 C8.1 | R31.2 26.8,59.05 26.8,60.45 35.56,60.45 v35.56,58.55 | v36.07,50.8 36.07,44.7
  Bottom 0.254: v35.56,58.55 36.07,58.55 v36.07,50.8
N$34  (via drill 0.6)
  Top 0.254: 2X_4IN_OR.13 v11.05,14.73 | v11.05,18.29 12.77,18.29 U$30.1 | v26.29,57.28 26.29,57.78 29.66,57.78
  Bottom 0.254: v11.05,14.73 v11.05,18.29 11.05,24.26 22.48,24.26 22.48,57.28 v26.29,57.28
N$41  (1 unrouted)
N$46  (1 unrouted)
N$47  (1 unrouted)
N$48  (1 unrouted)
RESET  (via drill 0.6)
  Top 0.254: 18.15,37.47 I2C_MULTIPLEXER.3 17.28,37.48 16.54,36.73 v15.21,36.73 | R21.1 v12.7,50.8
  Bottom 0.254: v15.21,36.73 15.21,46.99 12.7,46.99 v12.7,50.8
SCL_IN  (via drill 0.6)
  Top 0.254: 7.49,30.48 I2C.2 | v13.97,38.1 13.97,37.47 12.33,37.47 I2C_MULTIPLEXER.22 | v7.49,33.02 7.49,30.48 | 7.49,30.48 R20.1
  Bottom 0.254: v7.49,33.02 7.49,36.83 13.97,36.83 v13.97,38.1
SDA_IN  (via drill 0.6)
  Top 0.254: I2C.1 R19.1 | R19.1 7.94,28.26 | v11.43,35.2 11.43,36.83 I2C_MULTIPLEXER.23 | R19.1 7.87,27.94 v7.87,25.65
  Bottom 0.254: v11.43,35.2 11.43,33.02 v8.89,33.02 8.89,25.65 v7.87,25.65
VIB_0+  (1 unrouted)
  Top 0.254: U3.7 41.15,50.67 43.31,50.67 43.3,49.53 53.34,49.53
VIB_0-  (via drill 0.6)  (1 unrouted)
  Top 0.254: U3.9 40.14,50.67 38.35,50.67 v38.35,50.8 | v42.16,49.02 57.15,49.02
  Bottom 0.254: v42.16,49.02 42.16,49.53 38.35,49.53 v38.35,50.8
VIB_1+  (1 unrouted)
  Top 0.254: U1.7 47.5,53.47 44.45,53.47 44.45,55.88
VIB_1-  (1 unrouted)
  Top 0.254: U1.9 46.48,52.96 43.18,52.96

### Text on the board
tPlace: 3V3 | GND | 5V | 5V | Haptic PCB, Rev. 1 | E.A.S.I. | Project | University of Central Florida | SCL | SDA | S6 | S5 | S4 | S3 | S2 | S1 | S0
